| IBIS file stm32l0_51_52_53_62_63_ufqfn32.ibs
| Created by s2ibis version 1.1 (customized version)
| North Carolina State University, ERL, 2006
[IBIS ver] 4.2
[File name] stm32l0_51_52_53_62_63_ufqfn32.ibs
[File Rev] 1.0
[Date]  15-10-2014
[Source] Data Created at STMicroelectronics
[Notes]  File originated from ELDO simulations.
[Disclaimer]  This information is for modeling purpose only and is
   not guaranted. The information is subject to change without
   notice.
[Copyright] Copyright 2016 STMicroelectronics Inc.
|   Component stm32l0_51_52_53_62_63_ufqfn32
[Component] stm32l0_51_52_53_62_63_ufqfn32
[Manufacturer] STMicroelectronics
[Package]
| variable   typ   min   max
R_pkg   0.0   0.0   0.0
L_pkg   0.0H   0.0H   0.0H
C_pkg   0.0F   0.0F   0.0F
[Pin]  signal_name   model_name   R_pin   L_pin   C_pin
2 PC14-OSC32_IN io8p_wsudq_ls_ft_v33
3 PC15-OSC32_OUT io8p_sudq_ls_tc_esdft
4 NRST ioreset_tc_v33_esdft
5 VDDA POWER
6 PA0 io8p_wsudq_ls_ft_v33
7 PA1 io8p_wsudq_lcd4_ls_ft
8 PA2 io8p_wsudq_lcd4_ls_ft
9 PA3 io8p_wsudq_lcd4_ls_ft
10 PA4 io8p_wsudq_i2cin_ls_ft
11 PA5 io8p_wsudq_i2cin_ls_ft
12 PA6 io8p_wsudq_lcd4_ls_ft
13 PA7 io8p_wsudq_lcd4_ls_ft
14 PB0 io8p_wsudq_lcd4_ls_ft
15 PB1 io8p_wsudq_lcd4_ls_ft
16 PB2 io8p_wsudq_lcd4_ls_ft
17 VDD POWER
18 PA8 io8p_wsudq_lcd4_ls_ft
19 PA9 io8p_wsudq_lcd4_ls_ft
20 PA10 io8p_wsudq_lcd4_ls_ft
21 PA11 io8usb_ls_ft
22 PA12 io8usb_ls_ft
23 PA13 io8p_sudq_ls_ft
24 PA14 io8p_sudq_ls_ft
25 PA15 io8p_wsudq_lcd4_ls_ft
26 PB3 io8p_wsudq_lcd4_ls_ft
27 PB4 io8p_wsudq_lcd4_ls_ft
28 PB5 io8p_wsudq_lcd4_ls_ft
29 PB6 io8p_wsudq_i2cin_ls_ft
30 PB7 io8p_wsudq_i2cin_ls_ft
31 BOOT0 vpp_test_hv
32 PB8 io8p_sudq_lcd4_i2cin_ls_ft
1 VDD POWER
[Model Selector] io8p_sudq_ls_ft
io8p00_sudq_ls_ft_pd_lv  "SPEED00 1P8V, PD=40kOhm"
io8p00_sudq_ls_ft_pu_lv  "SPEED00 1P8V, PU=40kOhm"
io8p00_sudq_ls_ft_lv  "SPEED00 1P8V"
io8p01_sudq_ls_ft_pd_lv  "SPEED01 1P8V, PD=40kOhm"
io8p01_sudq_ls_ft_pu_lv  "SPEED01 1P8V, PU=40kOhm"
io8p01_sudq_ls_ft_lv  "SPEED01 1P8V"
io8p10_sudq_ls_ft_pd_lv  "SPEED10 1P8V, PD=40kOhm"
io8p10_sudq_ls_ft_pu_lv  "SPEED10 1P8V, PU=40kOhm"
io8p10_sudq_ls_ft_lv  "SPEED10 1P8V"
io8p11_sudq_ls_ft_pd_lv  "SPEED11 1P8V, PD=40kOhm"
io8p11_sudq_ls_ft_pu_lv  "SPEED11 1P8V, PU=40kOhm"
io8p11_sudq_ls_ft_lv  "SPEED11 1P8V"
io8p00_sudq_ls_ft_pd  "SPEED00, PD=40kOhm"
io8p00_sudq_ls_ft_pu  "SPEED00, PU=40kOhm"
io8p00_sudq_ls_ft  "SPEED00"
io8p01_sudq_ls_ft_pd  "SPEED01, PD=40kOhm"
io8p01_sudq_ls_ft_pu  "SPEED01, PU=40kOhm"
io8p01_sudq_ls_ft  "SPEED01"
io8p10_sudq_ls_ft_pd  "SPEED10, PD=40kOhm"
io8p10_sudq_ls_ft_pu  "SPEED10, PU=40kOhm"
io8p10_sudq_ls_ft  "SPEED10"
io8p11_sudq_ls_ft_pd  "SPEED11, PD=40kOhm"
io8p11_sudq_ls_ft_pu  "SPEED11, PU=40kOhm"
io8p11_sudq_ls_ft  "SPEED11"
[Model Selector] io8p_sudq_ls_tc_esdft
io8p00_sudq_ls_tc_esdft_pd_lv  "SPEED00 1P8V, PD=40kOhm"
io8p00_sudq_ls_tc_esdft_pu_lv  "SPEED00 1P8V, PU=40kOhm"
io8p00_sudq_ls_tc_esdft_lv  "SPEED00 1P8V"
io8p01_sudq_ls_tc_esdft_pd_lv  "SPEED01 1P8V, PD=40kOhm"
io8p01_sudq_ls_tc_esdft_pu_lv  "SPEED01 1P8V, PU=40kOhm"
io8p01_sudq_ls_tc_esdft_lv  "SPEED01 1P8V"
io8p10_sudq_ls_tc_esdft_pd_lv  "SPEED10 1P8V, PD=40kOhm"
io8p10_sudq_ls_tc_esdft_pu_lv  "SPEED10 1P8V, PU=40kOhm"
io8p10_sudq_ls_tc_esdft_lv  "SPEED10 1P8V"
io8p11_sudq_ls_tc_esdft_pd_lv  "SPEED11 1P8V, PD=40kOhm"
io8p11_sudq_ls_tc_esdft_pu_lv  "SPEED11 1P8V, PU=40kOhm"
io8p11_sudq_ls_tc_esdft_lv  "SPEED11 1P8V"
io8p00_sudq_ls_tc_esdft_pd  "SPEED00, PD=40kOhm"
io8p00_sudq_ls_tc_esdft_pu  "SPEED00, PU=40kOhm"
io8p00_sudq_ls_tc_esdft  "SPEED00"
io8p01_sudq_ls_tc_esdft_pd  "SPEED01, PD=40kOhm"
io8p01_sudq_ls_tc_esdft_pu  "SPEED01, PU=40kOhm"
io8p01_sudq_ls_tc_esdft  "SPEED01"
io8p10_sudq_ls_tc_esdft_pd  "SPEED10, PD=40kOhm"
io8p10_sudq_ls_tc_esdft_pu  "SPEED10, PU=40kOhm"
io8p10_sudq_ls_tc_esdft  "SPEED10"
io8p11_sudq_ls_tc_esdft_pd  "SPEED11, PD=40kOhm"
io8p11_sudq_ls_tc_esdft_pu  "SPEED11, PU=40kOhm"
io8p11_sudq_ls_tc_esdft  "SPEED11"
[Model Selector] io8p_wsudq_i2cin_ls_ft
io8p00_wsudq_i2cin_ls_ft_pd_lv  "SPEED00 1P8V, PD=40kOhm"
io8p00_wsudq_i2cin_ls_ft_pu_lv  "SPEED00 1P8V, PU=40kOhm"
io8p00_wsudq_i2cin_ls_ft_lv  "SPEED00 1P8V"
io8p01_wsudq_i2cin_ls_ft_pd_lv  "SPEED01 1P8V, PD=40kOhm"
io8p01_wsudq_i2cin_ls_ft_pu_lv  "SPEED01 1P8V, PU=40kOhm"
io8p01_wsudq_i2cin_ls_ft_lv  "SPEED01 1P8V"
io8p10_wsudq_i2cin_ls_ft_pd_lv  "SPEED10 1P8V, PD=40kOhm"
io8p10_wsudq_i2cin_ls_ft_pu_lv  "SPEED10 1P8V, PU=40kOhm"
io8p10_wsudq_i2cin_ls_ft_lv  "SPEED10 1P8V"
io8p11_wsudq_i2cin_ls_ft_pd_lv  "SPEED11 1P8V, PD=40kOhm"
io8p11_wsudq_i2cin_ls_ft_pu_lv  "SPEED11 1P8V, PU=40kOhm"
io8p11_wsudq_i2cin_ls_ft_lv  "SPEED11 1P8V"
io8p00_wsudq_i2cin_ls_ft_pd  "SPEED00, PD=40kOhm"
io8p00_wsudq_i2cin_ls_ft_pu  "SPEED00, PU=40kOhm"
io8p00_wsudq_i2cin_ls_ft  "SPEED00"
io8p01_wsudq_i2cin_ls_ft_pd  "SPEED01, PD=40kOhm"
io8p01_wsudq_i2cin_ls_ft_pu  "SPEED01, PU=40kOhm"
io8p01_wsudq_i2cin_ls_ft  "SPEED01"
io8p10_wsudq_i2cin_ls_ft_pd  "SPEED10, PD=40kOhm"
io8p10_wsudq_i2cin_ls_ft_pu  "SPEED10, PU=40kOhm"
io8p10_wsudq_i2cin_ls_ft  "SPEED10"
io8p11_wsudq_i2cin_ls_ft_pd  "SPEED11, PD=40kOhm"
io8p11_wsudq_i2cin_ls_ft_pu  "SPEED11, PU=40kOhm"
io8p11_wsudq_i2cin_ls_ft  "SPEED11"
[Model Selector] io8p_wsudq_lcd4_ls_ft
io8p00_wsudq_lcd4_ls_ft_pd_lv  "SPEED00 1P8V, PD=40kOhm"
io8p00_wsudq_lcd4_ls_ft_pu_lv  "SPEED00 1P8V, PU=40kOhm"
io8p00_wsudq_lcd4_ls_ft_lv  "SPEED00 1P8V"
io8p01_wsudq_lcd4_ls_ft_pd_lv  "SPEED01 1P8V, PD=40kOhm"
io8p01_wsudq_lcd4_ls_ft_pu_lv  "SPEED01 1P8V, PU=40kOhm"
io8p01_wsudq_lcd4_ls_ft_lv  "SPEED01 1P8V"
io8p10_wsudq_lcd4_ls_ft_pd_lv  "SPEED10 1P8V, PD=40kOhm"
io8p10_wsudq_lcd4_ls_ft_pu_lv  "SPEED10 1P8V, PU=40kOhm"
io8p10_wsudq_lcd4_ls_ft_lv  "SPEED10 1P8V"
io8p11_wsudq_lcd4_ls_ft_pd_lv  "SPEED11 1P8V, PD=40kOhm"
io8p11_wsudq_lcd4_ls_ft_pu_lv  "SPEED11 1P8V, PU=40kOhm"
io8p11_wsudq_lcd4_ls_ft_lv  "SPEED11 1P8V"
io8p00_wsudq_lcd4_ls_ft_pd  "SPEED00, PD=40kOhm"
io8p00_wsudq_lcd4_ls_ft_pu  "SPEED00, PU=40kOhm"
io8p00_wsudq_lcd4_ls_ft  "SPEED00"
io8p01_wsudq_lcd4_ls_ft_pd  "SPEED01, PD=40kOhm"
io8p01_wsudq_lcd4_ls_ft_pu  "SPEED01, PU=40kOhm"
io8p01_wsudq_lcd4_ls_ft  "SPEED01"
io8p10_wsudq_lcd4_ls_ft_pd  "SPEED10, PD=40kOhm"
io8p10_wsudq_lcd4_ls_ft_pu  "SPEED10, PU=40kOhm"
io8p10_wsudq_lcd4_ls_ft  "SPEED10"
io8p11_wsudq_lcd4_ls_ft_pd  "SPEED11, PD=40kOhm"
io8p11_wsudq_lcd4_ls_ft_pu  "SPEED11, PU=40kOhm"
io8p11_wsudq_lcd4_ls_ft  "SPEED11"
[Model Selector] io8p_wsudq_ls_ft_v33
io8p00_wsudq_ls_ft_v33_pd_lv  "SPEED00 1P8V, PD=40kOhm"
io8p00_wsudq_ls_ft_v33_pu_lv  "SPEED00 1P8V, PU=40kOhm"
io8p00_wsudq_ls_ft_v33_lv  "SPEED00 1P8V"
io8p01_wsudq_ls_ft_v33_pd_lv  "SPEED01 1P8V, PD=40kOhm"
io8p01_wsudq_ls_ft_v33_pu_lv  "SPEED01 1P8V, PU=40kOhm"
io8p01_wsudq_ls_ft_v33_lv  "SPEED01 1P8V"
io8p10_wsudq_ls_ft_v33_pd_lv  "SPEED10 1P8V, PD=40kOhm"
io8p10_wsudq_ls_ft_v33_pu_lv  "SPEED10 1P8V, PU=40kOhm"
io8p10_wsudq_ls_ft_v33_lv  "SPEED10 1P8V"
io8p11_wsudq_ls_ft_v33_pd_lv  "SPEED11 1P8V, PD=40kOhm"
io8p11_wsudq_ls_ft_v33_pu_lv  "SPEED11 1P8V, PU=40kOhm"
io8p11_wsudq_ls_ft_v33_lv  "SPEED11 1P8V"
io8p00_wsudq_ls_ft_v33_pd  "SPEED00, PD=40kOhm"
io8p00_wsudq_ls_ft_v33_pu  "SPEED00, PU=40kOhm"
io8p00_wsudq_ls_ft_v33  "SPEED00"
io8p01_wsudq_ls_ft_v33_pd  "SPEED01, PD=40kOhm"
io8p01_wsudq_ls_ft_v33_pu  "SPEED01, PU=40kOhm"
io8p01_wsudq_ls_ft_v33  "SPEED01"
io8p10_wsudq_ls_ft_v33_pd  "SPEED10, PD=40kOhm"
io8p10_wsudq_ls_ft_v33_pu  "SPEED10, PU=40kOhm"
io8p10_wsudq_ls_ft_v33  "SPEED10"
io8p11_wsudq_ls_ft_v33_pd  "SPEED11, PD=40kOhm"
io8p11_wsudq_ls_ft_v33_pu  "SPEED11, PU=40kOhm"
io8p11_wsudq_ls_ft_v33  "SPEED11"
[Model Selector] ioreset_tc_v33_esdft
ioreset_tc_v33_esdft_pu_lv  "IORESET 1P65V + PU=40kOhm"
ioreset_tc_v33_esdft_nopu_lv  "IORESET 1P65V"
ioreset_tc_v33_esdft_pu  "IORESET + PU=40kOhm"
ioreset_tc_v33_esdft_nopu  "IORESET"
[Model Selector] vpp_test_hv
vpp_test_hv_2p4  "Input Buffer 1P65V"
vpp_test_hv_3p3  "Input Buffer"
[Model Selector] io8usb_ls_ft
io8usb_ls_ft_dpdn_pu  "HS USB DP/DN IO + PU=1.2kOhm"
io8usb_ls_ft_dpdn  "HS USB DP/DN IO"
io8p00_ls_ft_pd_lv  "SPEED00 1P8V, PD=40kOhm"
io8p00_ls_ft_pu_lv  "SPEED00 1P8V, PU=40kOhm"
io8p00_ls_ft_lv  "SPEED00 1P8V"
io8p01_ls_ft_pd_lv  "SPEED01 1P8V, PD=40kOhm"
io8p01_ls_ft_pu_lv  "SPEED01 1P8V, PU=40kOhm"
io8p01_ls_ft_lv  "SPEED01 1P8V"
io8p10_ls_ft_pd_lv  "SPEED10 1P8V, PD=40kOhm"
io8p10_ls_ft_pu_lv  "SPEED10 1P8V, PU=40kOhm"
io8p10_ls_ft_lv  "SPEED10 1P8V"
io8p11_ls_ft_pd_lv  "SPEED11 1P8V, PD=40kOhm"
io8p11_ls_ft_pu_lv  "SPEED11 1P8V, PU=40kOhm"
io8p11_ls_ft_lv  "SPEED11 1P8V"
io8p00_ls_ft_pd  "SPEED00, PD=40kOhm"
io8p00_ls_ft_pu  "SPEED00, PU=40kOhm"
io8p00_ls_ft  "SPEED00"
io8p01_ls_ft_pd  "SPEED01, PD=40kOhm"
io8p01_ls_ft_pu  "SPEED01, PU=40kOhm"
io8p01_ls_ft  "SPEED01"
io8p10_ls_ft_pd  "SPEED10, PD=40kOhm"
io8p10_ls_ft_pu  "SPEED10, PU=40kOhm"
io8p10_ls_ft  "SPEED10"
io8p11_ls_ft_pd  "SPEED11, PD=40kOhm"
io8p11_ls_ft_pu  "SPEED11, PU=40kOhm"
io8p11_ls_ft  "SPEED11"
[Model Selector] io8p_sudq_lcd4_i2cin_ls_ft
io8p00_sudq_lcd4_i2cin_ls_ft_pd_lv  "SPEED00 1P8V, PD=40kOhm"
io8p00_sudq_lcd4_i2cin_ls_ft_pu_lv  "SPEED00 1P8V, PU=40kOhm"
io8p00_sudq_lcd4_i2cin_ls_ft_lv  "SPEED00 1P8V"
io8p01_sudq_lcd4_i2cin_ls_ft_pd_lv  "SPEED01 1P8V, PD=40kOhm"
io8p01_sudq_lcd4_i2cin_ls_ft_pu_lv  "SPEED01 1P8V, PU=40kOhm"
io8p01_sudq_lcd4_i2cin_ls_ft_lv  "SPEED01 1P8V"
io8p10_sudq_lcd4_i2cin_ls_ft_pd_lv  "SPEED10 1P8V, PD=40kOhm"
io8p10_sudq_lcd4_i2cin_ls_ft_pu_lv  "SPEED10 1P8V, PU=40kOhm"
io8p10_sudq_lcd4_i2cin_ls_ft_lv  "SPEED10 1P8V"
io8p11_sudq_lcd4_i2cin_ls_ft_pd_lv  "SPEED11 1P8V, PD=40kOhm"
io8p11_sudq_lcd4_i2cin_ls_ft_pu_lv  "SPEED11 1P8V, PU=40kOhm"
io8p11_sudq_lcd4_i2cin_ls_ft_lv  "SPEED11 1P8V"
io8p00_sudq_lcd4_i2cin_ls_ft_pd  "SPEED00, PD=40kOhm"
io8p00_sudq_lcd4_i2cin_ls_ft_pu  "SPEED00, PU=40kOhm"
io8p00_sudq_lcd4_i2cin_ls_ft  "SPEED00"
io8p01_sudq_lcd4_i2cin_ls_ft_pd  "SPEED01, PD=40kOhm"
io8p01_sudq_lcd4_i2cin_ls_ft_pu  "SPEED01, PU=40kOhm"
io8p01_sudq_lcd4_i2cin_ls_ft  "SPEED01"
io8p10_sudq_lcd4_i2cin_ls_ft_pd  "SPEED10, PD=40kOhm"
io8p10_sudq_lcd4_i2cin_ls_ft_pu  "SPEED10, PU=40kOhm"
io8p10_sudq_lcd4_i2cin_ls_ft  "SPEED10"
io8p11_sudq_lcd4_i2cin_ls_ft_pd  "SPEED11, PD=40kOhm"
io8p11_sudq_lcd4_i2cin_ls_ft_pu  "SPEED11, PU=40kOhm"
io8p11_sudq_lcd4_i2cin_ls_ft  "SPEED11"
| Models and submodels in the file (176): io8p00_sudq_ls_ft_pd_lv (I/O), io8p00_sudq_ls_ft_pu_lv (I/O), io8p00_sudq_ls_ft_lv (I/O), io8p01_sudq_ls_ft_pd_lv (I/O), io8p01_sudq_ls_ft_pu_lv (I/O), io8p01_sudq_ls_ft_lv (I/O), io8p10_sudq_ls_ft_pd_lv (I/O), io8p10_sudq_ls_ft_pu_lv (I/O), io8p10_sudq_ls_ft_lv (I/O), io8p11_sudq_ls_ft_pd_lv (I/O), io8p11_sudq_ls_ft_pu_lv (I/O), io8p11_sudq_ls_ft_lv (I/O), io8p00_sudq_ls_ft_pd (I/O), io8p00_sudq_ls_ft_pu (I/O), io8p00_sudq_ls_ft (I/O), io8p01_sudq_ls_ft_pd (I/O), io8p01_sudq_ls_ft_pu (I/O), io8p01_sudq_ls_ft (I/O), io8p10_sudq_ls_ft_pd (I/O), io8p10_sudq_ls_ft_pu (I/O), io8p10_sudq_ls_ft (I/O), io8p11_sudq_ls_ft_pd (I/O), io8p11_sudq_ls_ft_pu (I/O), io8p11_sudq_ls_ft (I/O), io8p00_sudq_ls_tc_esdft_pd_lv (I/O), io8p00_sudq_ls_tc_esdft_pu_lv (I/O), io8p00_sudq_ls_tc_esdft_lv (I/O), io8p01_sudq_ls_tc_esdft_pd_lv (I/O), io8p01_sudq_ls_tc_esdft_pu_lv (I/O), io8p01_sudq_ls_tc_esdft_lv (I/O), io8p10_sudq_ls_tc_esdft_pd_lv (I/O), io8p10_sudq_ls_tc_esdft_pu_lv (I/O), io8p10_sudq_ls_tc_esdft_lv (I/O), io8p11_sudq_ls_tc_esdft_pd_lv (I/O), io8p11_sudq_ls_tc_esdft_pu_lv (I/O), io8p11_sudq_ls_tc_esdft_lv (I/O), io8p00_sudq_ls_tc_esdft_pd (I/O), io8p00_sudq_ls_tc_esdft_pu (I/O), io8p00_sudq_ls_tc_esdft (I/O), io8p01_sudq_ls_tc_esdft_pd (I/O), io8p01_sudq_ls_tc_esdft_pu (I/O), io8p01_sudq_ls_tc_esdft (I/O), io8p10_sudq_ls_tc_esdft_pd (I/O), io8p10_sudq_ls_tc_esdft_pu (I/O), io8p10_sudq_ls_tc_esdft (I/O), io8p11_sudq_ls_tc_esdft_pd (I/O), io8p11_sudq_ls_tc_esdft_pu (I/O), io8p11_sudq_ls_tc_esdft (I/O), io8p00_wsudq_i2cin_ls_ft_pd_lv (I/O), io8p00_wsudq_i2cin_ls_ft_pu_lv (I/O), io8p00_wsudq_i2cin_ls_ft_lv (I/O), io8p01_wsudq_i2cin_ls_ft_pd_lv (I/O), io8p01_wsudq_i2cin_ls_ft_pu_lv (I/O), io8p01_wsudq_i2cin_ls_ft_lv (I/O), io8p10_wsudq_i2cin_ls_ft_pd_lv (I/O), io8p10_wsudq_i2cin_ls_ft_pu_lv (I/O), io8p10_wsudq_i2cin_ls_ft_lv (I/O), io8p11_wsudq_i2cin_ls_ft_pd_lv (I/O), io8p11_wsudq_i2cin_ls_ft_pu_lv (I/O), io8p11_wsudq_i2cin_ls_ft_lv (I/O), io8p00_wsudq_i2cin_ls_ft_pd (I/O), io8p00_wsudq_i2cin_ls_ft_pu (I/O), io8p00_wsudq_i2cin_ls_ft (I/O), io8p01_wsudq_i2cin_ls_ft_pd (I/O), io8p01_wsudq_i2cin_ls_ft_pu (I/O), io8p01_wsudq_i2cin_ls_ft (I/O), io8p10_wsudq_i2cin_ls_ft_pd (I/O), io8p10_wsudq_i2cin_ls_ft_pu (I/O), io8p10_wsudq_i2cin_ls_ft (I/O), io8p11_wsudq_i2cin_ls_ft_pd (I/O), io8p11_wsudq_i2cin_ls_ft_pu (I/O), io8p11_wsudq_i2cin_ls_ft (I/O), io8p00_wsudq_lcd4_ls_ft_pd_lv (I/O), io8p00_wsudq_lcd4_ls_ft_pu_lv (I/O), io8p00_wsudq_lcd4_ls_ft_lv (I/O), io8p01_wsudq_lcd4_ls_ft_pd_lv (I/O), io8p01_wsudq_lcd4_ls_ft_pu_lv (I/O), io8p01_wsudq_lcd4_ls_ft_lv (I/O), io8p10_wsudq_lcd4_ls_ft_pd_lv (I/O), io8p10_wsudq_lcd4_ls_ft_pu_lv (I/O)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
